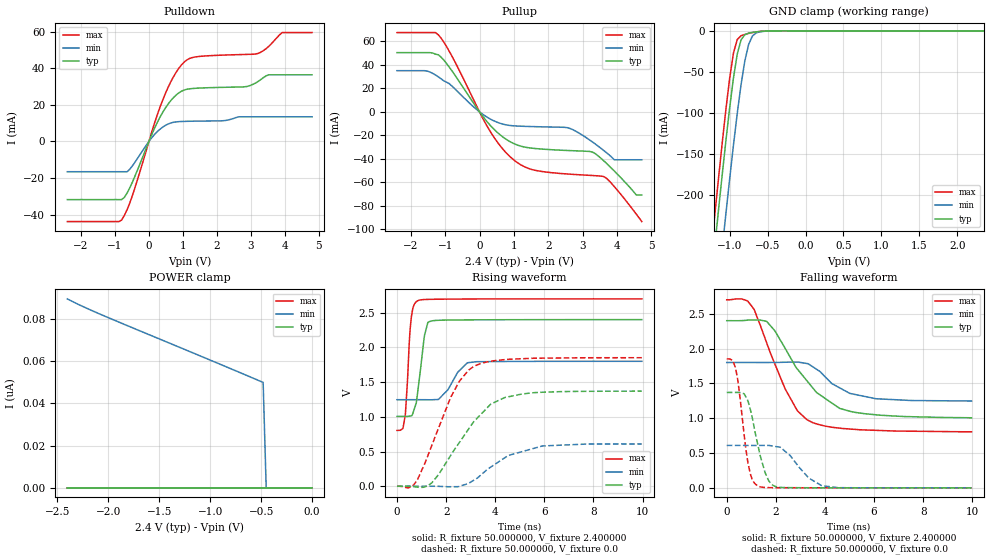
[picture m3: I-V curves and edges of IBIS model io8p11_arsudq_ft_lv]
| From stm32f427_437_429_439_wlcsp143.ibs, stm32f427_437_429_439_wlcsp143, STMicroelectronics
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|   Model io8p11_arsudq_ft_lv
[Model]  io8p11_arsudq_ft_lv
Model_type I/O
Polarity   Non-Inverting
Enable   Active-Low
Vinl =   0.720000V
Vinh =   1.680000V
Vmeas =  1.200000V
Cref =   30.000000pF
Rref =   100.000000M
Vref =   0.0V
C_comp   2.239000pF   2.178700pF   2.334000pF
[Temperature Range]   25.000000   0.125000k   -40.000000
[Pullup Reference]   2.400000V   1.800000V   2.700000V
[Pulldown Reference]   0.0V   0.0V   0.0V
[POWER Clamp Reference]   2.400000V   1.800000V   2.700000V
[GND Clamp Reference]   0.0V   0.0V   0.0V
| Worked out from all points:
|   slope of the pulldown table from 0 to 0.36 V, typ, clamps not added: 25 ohm
|   slope of the pullup table from 0 to 0.36 V, typ, clamps not added: 27.7 ohm
|   GND clamp passes 1 mA (typ) near -0.62 V on its own axis
|   rising waveform, R_fixture 50.000000, V_fixture 2.400000: 20-80 % time 281ps typ, 623ps min, 184ps max; typ from 1.01 V to 2.4 V
|   rising waveform, R_fixture 50.000000, V_fixture 0.0: 20-80 % time 1.7ns typ, 1.69ns min, 1.31ns max; typ from 0 V to 1.37 V
|   falling waveform, R_fixture 50.000000, V_fixture 2.400000: 20-80 % time 1.82ns typ, 1.29ns min, 1.38ns max; typ from 2.4 V to 1.01 V
|   falling waveform, R_fixture 50.000000, V_fixture 0.0: 20-80 % time 535ps typ, 925ps min, 383ps max; typ from 1.37 V to 0 V
[Pulldown]
|Voltage   I(typ)   I(min)   I(max)
-2.4V     -31.73mA   -16.51mA   -43.74mA
-800mV    -31.73mA   -16.51mA   -42.87mA
-480mV    -21.98mA   -13.17mA   -29.21mA
80mV      3.63mA     1.966mA    5.014mA
480mV     18.16mA    8.738mA    26.02mA
800mV     25.38mA    10.72mA    37.77mA
1.12V     28.53mA    11.02mA    44.6mA
2.8V      29.84mA    13.49mA    47.53mA
3.2V      32.65mA    13.49mA    48.05mA
3.52V     36.43mA    13.49mA    51.84mA
3.92V     36.43mA    13.49mA    59.49mA
4.8V      36.43mA    13.49mA    59.49mA
[Pullup]
|Voltage   I(typ)   I(min)   I(max)
-2.4V     50.45mA    35.08mA    67.53mA
-1.52V    50.45mA    34.74mA    67.53mA
-1.2V     48.64mA    29.87mA    65.68mA
320mV     -11.75mA   -6.207mA   -17.08mA
1.04V     -27.54mA   -11.97mA   -41.91mA
1.6V      -31.14mA   -12.58mA   -49.63mA
2.56V     -32.88mA   -13.48mA   -52.9mA
3.28V     -34.19mA   -25.52mA   -54.18mA
3.6V      -41.31mA   -32.62mA   -54.97mA
3.92V     -50.32mA   -40.8mA    -63.62mA
4.56V     -70.8mA    -40.8mA    -87.08mA
4.72V     -70.8mA    -40.8mA    -93.4mA
[GND_clamp]
|Voltage   I(typ)   I(min)   I(max)
-2.4V     -1.424A    -1.508A    -1.393A
-1.25V    -311.2mA   -401.9mA   -273.3mA
-1.2V     -265.4mA   -356.1mA   -227.2mA
-1.15V    -220.4mA   -310.8mA   -181.9mA
-1.1V     -176.3mA   -266.2mA   -137.9mA
-1.05V    -133.8mA   -222.5mA   -95.87mA
-950mV    -57.3mA    -138.9mA   -26.98mA
-900mV    -28.27mA   -100.4mA   -10.59mA
-850mV    -11.01mA   -65.54mA   -5.958mA
-750mV    -2.834mA   -16.5mA    -3.178mA
-600mV    -750uA     -1.164mA   -738.3uA
2.35V     0A         0A         0A
[POWER_clamp]
|Voltage   I(typ)   I(min)   I(max)
-2.4V     0A         89.62nA    0A
-2.04V    0A         81.57nA    0A
-480mV    0A         50.01nA    0A
-450mV    0A         0A         0A
0V        0A         0A         0A
[Ramp]
| variable   typ   min   max
dV/dt_r  0.82182/1.69447n   0.36401/1.67899n   1.11120/1.31075n
dV/dt_f  0.83262/1.81412n   0.33282/1.29832n   1.13582/1.37480n
R_load = 50.000000
[Rising Waveform]
R_fixture= 50.000000
V_fixture= 2.400000
V_fixture_min= 1.800000
V_fixture_max= 2.700000
|time   V(typ)   V(min)   V(max)
0s        1.006V     1.247V     804.6mV
240.2ps   1.006V     1.247V     832mV
340.3ps   1.006V     1.247V     1.038V
500.5ps   1.01V      1.247V     2.08V
580.6ps   1.015V     1.247V     2.428V
840.8ps   1.352V     1.247V     2.672V
1.121ns   2.176V     1.247V     2.69V
1.361ns   2.377V     1.245V     2.693V
2.883ns   2.397V     1.779V     2.697V
9.97ns    2.4V       1.8V       2.699V
[Rising Waveform]
R_fixture= 50.000000
V_fixture= 0.0
V_fixture_min= 0.0
V_fixture_max= 0.0
|time   V(typ)   V(min)   V(max)
0s        169.6uV    66.23uV    557.2uV
680.7ps   -5.47mV    52.05uV    19.57mV
1.421ns   50.63mV    101.3uV    592.1mV
2.202ns   453.5mV    -7.022mV   1.291V
2.543ns   632.3mV    -994.7uV   1.514V
3.143ns   936.2mV    90.72mV    1.729V
3.824ns   1.185V     278.2mV    1.8V
4.384ns   1.277V     409.3mV    1.824V
5.926ns   1.354V     580.5mV    1.845V
9.97ns    1.37V      609mV      1.852V
[Falling Waveform]
R_fixture= 50.000000
V_fixture= 2.400000
V_fixture_min= 1.800000
V_fixture_max= 2.700000
|time   V(typ)   V(min)   V(max)
0s        2.4V       1.8V       2.699V
660.7ps   2.402V     1.8V       2.707V
1.101ns   2.41V      1.8V       2.569V
1.622ns   2.391V     1.8V       2.087V
2.382ns   2.002V     1.803V     1.419V
2.883ns   1.703V     1.805V     1.104V
3.263ns   1.539V     1.785V     979.8mV
3.664ns   1.367V     1.702V     917.7mV
5.045ns   1.097V     1.354V     843.8mV
9.97ns    1.006V     1.247V     804.6mV
[Falling Waveform]
R_fixture= 50.000000
V_fixture= 0.0
V_fixture_min= 0.0
V_fixture_max= 0.0
|time   V(typ)   V(min)   V(max)
0s        1.37V      609mV      1.852V
360.4ps   1.37V      609mV      1.719V
460.5ps   1.37V      609mV      1.524V
720.7ps   1.345V     608.9mV    729.8mV
961ps     1.124V     608.7mV    200.3mV
1.281ns   594.4mV    608.7mV    26.29mV
1.702ns   107.4mV    609.8mV    3.567mV
2.062ns   12.48mV    589.9mV    2.327mV
3.884ns   1.066mV    29.55mV    1.165mV
9.97ns    169.6uV    66.23uV    557.2uV
